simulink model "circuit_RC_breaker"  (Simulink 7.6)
settings: Solver=ode23t  StartTime=0.0  StopTime=12  RelTol=1e-3
PreLoadFcn:
  | close all
  | clc
  | clear all
StopFcn:
  | close all
  | load tension_Vc.mat
  | plotyy(x(1,:),x(2,:),x(1,:),x(3,:))
  | grid
  | title('Tension aux bornes du condensateur C- Commande du Breaker')
  | xlabel('temps')
undefined symbols (not defined in the file or in its folder): sigbuilder_block
libraries: powerlib x10

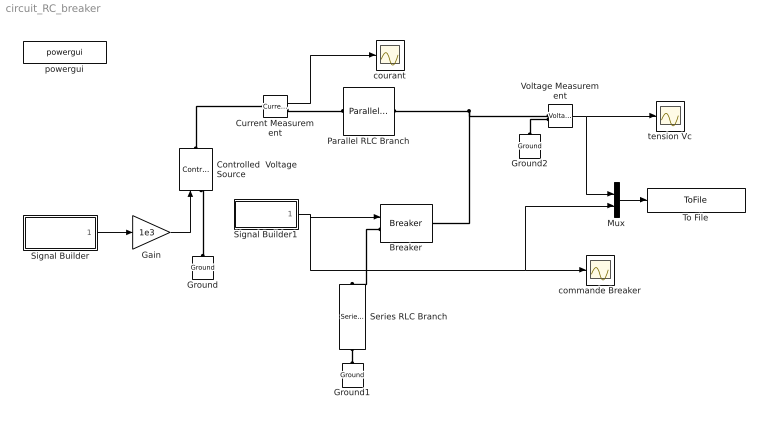
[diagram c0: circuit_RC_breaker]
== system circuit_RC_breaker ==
  Breaker : powerlib/Elements/Breaker  DialogController=POWERSYS.PowerSysDialog  SystemSampleTime=-1  BreakerResistance=0.0001  InitialState=0  SnubberResistance=1e6  SnubberCapacitance=inf  SwitchingTimes="[ 1/60  5/60 ]"  External=on  Measurements=None  MoreParameters=off  NoBreakLoop=off
  Controlled  Voltage Source : powerlib/Electrical Sources/Controlled Voltage Source  DialogController=POWERSYS.PowerSysDialog  SystemSampleTime=-1  Initialize=on  Source_Type=AC  Amplitude=0  Phase=0  Frequency=0  Measurements=None
  Current Measurement : powerlib/Measurements/Current Measurement  DialogController=POWERSYS.PowerSysDialog  SystemSampleTime=-1  PhasorSimulation=off  OutputType=Complex  PSBequivalent=0
  Gain : Gain  Gain=1e3
  Ground : powerlib/Elements/Ground  DialogController=POWERSYS.PowerSysDialog  PhysicalDomain=powersysdomain  SubClassName=unknown  LeftPortType=p1  RightPortType=p1  LConnTagsString=a
  Ground1 : powerlib/Elements/Ground  DialogController=POWERSYS.PowerSysDialog  PhysicalDomain=powersysdomain  SubClassName=unknown  LeftPortType=p1  RightPortType=p1  LConnTagsString=a
  Ground2 : powerlib/Elements/Ground  DialogController=POWERSYS.PowerSysDialog  PhysicalDomain=powersysdomain  SubClassName=unknown  LeftPortType=p1  RightPortType=p1  LConnTagsString=a
  Mux : Mux  Inputs=2
  Parallel RLC Branch : powerlib/Elements/Parallel RLC Branch  DialogController=POWERSYS.PowerSysDialog  PhysicalDomain=powersysdomain  SubClassName=unknown  LeftPortType=p1  RightPortType=p1  LConnTagsString=a  RConnTagsString=__new0  BranchType=R  Resistance=1000  Inductance=1e-3  SetiL0=off  InitialCurrent=0  Capacitance=1e-6  Setx0=off  InitialVoltage=0  Measurements=None
  Series RLC Branch : powerlib/Elements/Series RLC Branch  DialogController=POWERSYS.PowerSysDialog  PhysicalDomain=powersysdomain  SubClassName=unknown  LeftPortType=p1  RightPortType=p1  LConnTagsString=__new0  RConnTagsString=__new0  BranchType=RLC  Resistance=0  Inductance=0  SetiL0=off  InitialCurrent=0  Capacitance=0.001  Setx0=off  InitialVoltage=0  Measurements=None
  Signal Builder : Subsystem  Tag=STV Subsys  LoadFcn=sigbuilder_block('load');  StartFcn=sigbuilder_block('start');  StopFcn=sigbuilder_block('stop');  ClipboardFcn=sigbuilder_block('clipboard');
  Signal Builder1 : Subsystem  Tag=STV Subsys  LoadFcn=sigbuilder_block('load');  StartFcn=sigbuilder_block('start');  StopFcn=sigbuilder_block('stop');  ClipboardFcn=sigbuilder_block('clipboard');
  To File : ToFile  Filename=tension_Vc.mat  MatrixName=x
  Voltage Measurement : powerlib/Measurements/Voltage Measurement  DialogController=POWERSYS.PowerSysDialog  SystemSampleTime=-1  PhasorSimulation=off  OutputType=Complex  PSBequivalent=0
  commande Breaker : Scope
  courant : Scope
  powergui : powerlib/powergui  SystemSampleTime=-1  SimulationMode=Continuous  SampleTime=0  frequency=60  SPID=off  DisableSnubberDevices=off  DisableRonSwitches=off  DisableVfSwitches=off  SwTol=0  Interpol=off  frequencyindice=0  echomessages=off  HookPort=off  DisplayEquations=off  FunctionMessages=off  EnableUseOfTLC=off  x0status=blocks  RestoreLinks=warning  ResistiveCurrentMeasurement=off  Frange=[0:2:500]  Ylog=off  Xlog=on  ShowGrid=off  save=off  variable=ZData  ZoomFFT=on  StartTime=0.0  cycles=1  DisplayStyle=1  fundamental=60  FreqAxis=off  MaxFrequency=1000  frequencyindicesteady=1  RmsSteady=1  display=off  Ts=0  methode=off
  tension Vc : Scope
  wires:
  Current Measurement/1 -> courant/1
  Voltage Measurement/1 -> tension Vc/1, Mux/1
  Mux/1 -> To File/1
  Signal Builder/1(Signal 1) -> Gain/1
  Gain/1 -> Controlled  Voltage Source/1
  Signal Builder1/1(Signal 2) -> Mux/2, commande Breaker/1, Breaker/1
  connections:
  Ground/LConn1 -- Controlled  Voltage Source/LConn1
  Controlled  Voltage Source/RConn1 -- Current Measurement/LConn1
  Current Measurement/RConn1 -- Parallel RLC Branch/LConn1
  Ground2/LConn1 -- Voltage Measurement/LConn2
  Parallel RLC Branch/RConn1 -- Voltage Measurement/LConn1 -- Breaker/RConn1
  Breaker/LConn1 -- Series RLC Branch/LConn1
  Series RLC Branch/RConn1 -- Ground1/LConn1

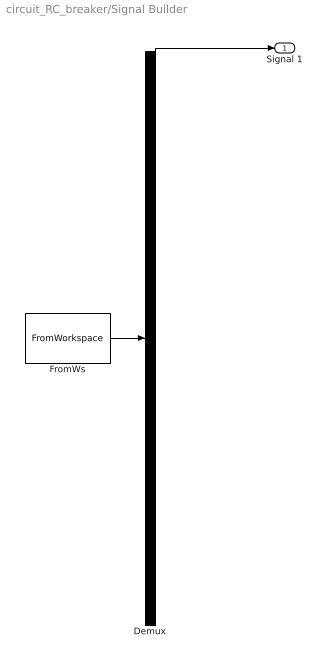
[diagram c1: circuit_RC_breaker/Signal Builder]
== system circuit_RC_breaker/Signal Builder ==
  Demux : Demux  Tag=STV Demux  Outputs=1
  FromWs : FromWorkspace  Tag=STV FromWs  VariableName=tuvar  SampleTime=0  SigBuilderData=DataTag0  VnvData=DataTag1
  Signal 1 : Outport  Tag=STV Outport
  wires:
  FromWs/1 -> Demux/1
  Demux/1 -> Signal 1/1

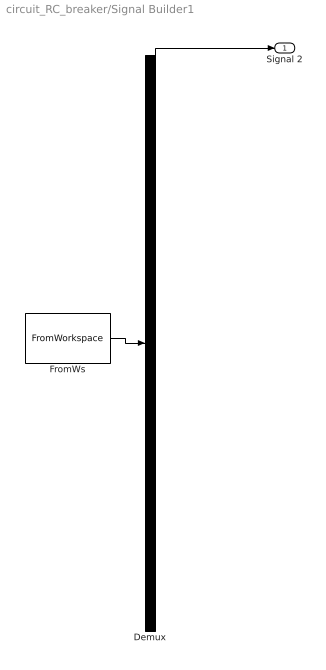
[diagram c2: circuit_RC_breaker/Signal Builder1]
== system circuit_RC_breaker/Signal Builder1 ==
  Demux : Demux  Tag=STV Demux  Outputs=1
  FromWs : FromWorkspace  Tag=STV FromWs  VariableName=tuvar  SampleTime=0  SigBuilderData=DataTag2  VnvData=DataTag3
  Signal 2 : Outport  Tag=STV Outport
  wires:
  FromWs/1 -> Demux/1
  Demux/1 -> Signal 2/1
